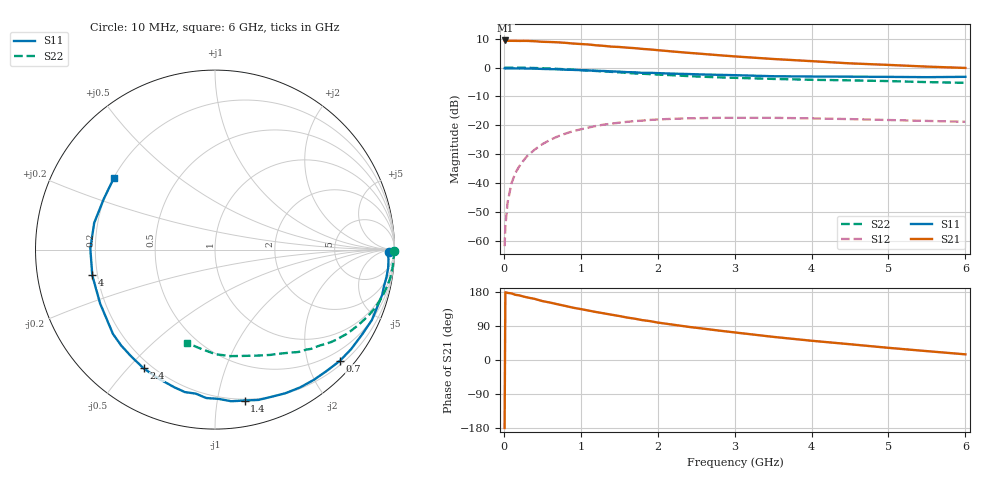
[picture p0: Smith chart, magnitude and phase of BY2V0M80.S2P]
! SIEMENS Small Signal Semiconductors
! BFY420
! Si NPN RF SIEGET Grounded Emitter Transistor in MICRO-X
! VCE = 2 V  IC = 0.8 mA
! Common Emitter S-Parameters:  October  1996
# GHz  S  MA  R  50
!  f  S11  S21  S12  S22
! GHz  MAG  ANG  MAG  ANG  MAG  ANG  MAG  ANG
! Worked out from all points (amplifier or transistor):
!   36 points, 10 MHz to 6 GHz, reference 50 ohm
!   highest |S21| = 9.4 dB at 20 MHz (marker M1)
!   |S21| within 3 dB of that: start of sweep to 1.84 GHz
!   unconditionally stable (mu >= 1): 4.647 GHz to end of sweep
!   at 250 MHz: K = 0.03, MSG = 20.8 dB, |S12| = -32.4 dB
!   at 1.4 GHz: K = 0.19, MSG = 13.4 dB, |S12| = -19.5 dB
!   at 6 GHz: K = 1.37, MAG = 5.7 dB, |S12| = -18.8 dB
!   S11 on the Smith chart (normalised r, x): 10 MHz: 53, -28; 700 MHz: 0.28, -2.60; 1.4 GHz: 0.19, -1.20; 2.4 GHz: 0.17, -0.55; 4 GHz: 0.18, -0.10; 6 GHz: 0.20, +0.31
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0.01  0.971 -0.9  2.947 -179.4  0.0008 102.4  0.999 -0.3
0.02  0.9621 -1.4  2.949 178.8  0.0018 94.5  0.9965 -0.5
0.05  0.9682 -3.1  2.907 177.1  0.0047 83.5  0.998 -1.5
0.1  0.9702 -6.1  2.904 175.7  0.0099 87.3  0.9956 -3.0
0.15  0.9676 -9.2  2.903 172.1  0.0149 84.0  0.9947 -4.5
0.3  0.9603 -18.0  2.897 165.3  0.0289 78.8  0.9896 -8.9
0.4  0.958 -24.2  2.86 161.3  0.0377 75.3  0.9819 -11.8
0.5  0.9459 -30.2  2.797 155.5  0.0469 71.4  0.9714 -14.7
0.7  0.9319 -41.7  2.738 147.0  0.0639 64.3  0.9474 -20.3
0.9  0.911 -52.8  2.609 138.0  0.0789 57.2  0.9168 -25.4
1.1  0.8912 -63.9  2.512 130.5  0.091 50.8  0.8866 -30.2
1.4  0.857 -78.9  2.304 119.5  0.1064 42.1  0.8412 -36.7
1.7  0.8283 -93.4  2.169 109.1  0.1178 34.2  0.7912 -42.5
2  0.8 -106.4  2.002 98.8  0.1259 27.4  0.7552 -47.5
2.2  0.7843 -113.8  1.896 93.2  0.1293 23.2  0.7353 -50.9
2.4  0.7717 -121.0  1.8 87.5  0.1316 19.7  0.7104 -53.9
2.8  0.7476 -134.3  1.634 77.5  0.1344 13.2  0.6754 -59.4
3.5  0.7071 -154.8  1.408 61.1  0.1344 4.6  0.6353 -68.4
4  0.6986 -168.2  1.291 50.8  0.1314 -0.1  0.6134 -74.9
4.5  0.6946 179.5  1.182 41.6  0.1277 -4.0  0.5997 -81.8
5.5  0.6811 155.6  1.038 23.4  0.1188 -7.5  0.5591 -97.7
6  0.6905 144.6  0.984 14.9  0.1147 -7.2  0.5429 -106.6
